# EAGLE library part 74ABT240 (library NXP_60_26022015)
Octal BUFFER and LINE DRIVER, 3-state
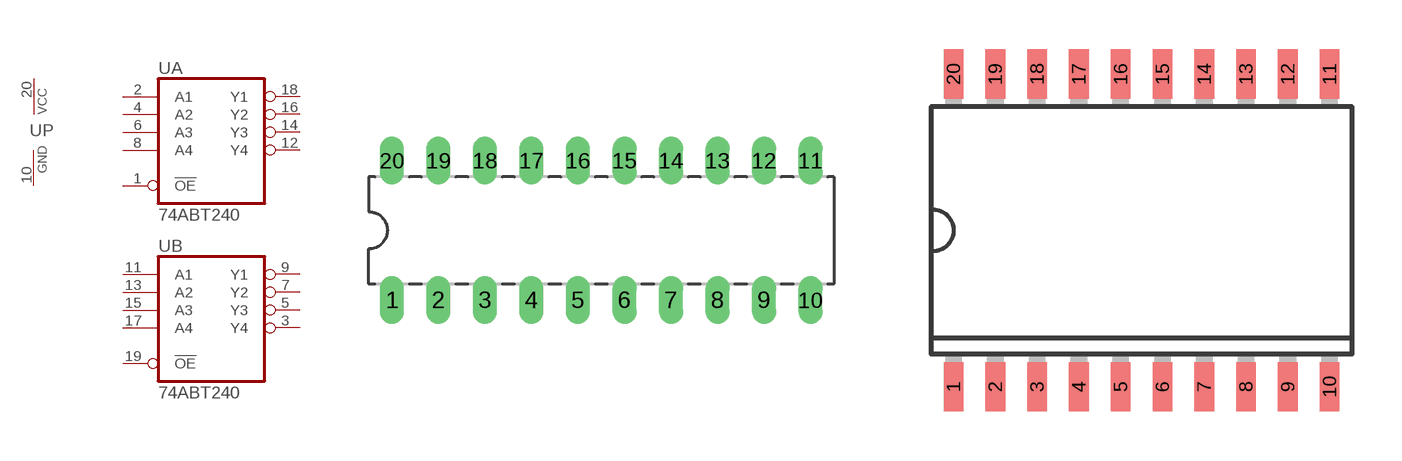
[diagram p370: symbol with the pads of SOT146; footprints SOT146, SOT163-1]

Designator prefix U; gates A=74240 B=74240 P=PWRN-3

## 74ABT240N  [SOT146]
1  A:!OE  in
2  A:A1  in
3  B:Y4  hiz
4  A:A2  in
5  B:Y3  hiz
6  A:A3  in
7  B:Y2  hiz
8  A:A4  in
9  B:Y1  hiz
10  P:GND  pwr
11  B:A1  in
12  A:Y4  hiz
13  B:A2  in
14  A:Y3  hiz
15  B:A3  in
16  A:Y2  hiz
17  B:A4  in
18  A:Y1  hiz
19  B:!OE  in
20  P:VCC  pwr

## 74ABT240D  [SOT163-1]
Pads as for SOT146

## 74ABT240DB  [SOT339]
Pads as for SOT146

## 74ABT240PW  [SOT360]
Pads as for SOT146

## Footprint SOT146 (pad centres in mm)
SOT146 DIP20: plastic dual in-line package; 20 leads (300 mil) JEDEC: MS-001 IEC: -- JEITA: SC-603
drill 0.813 long: 1 -11.43,-3.81; 2 -8.89,-3.81; 3 -6.35,-3.81; 4 -3.81,-3.81; 5 -1.27,-3.81; 6 1.27,-3.81; 7 3.81,-3.81; 8 6.35,-3.81; 9 8.89,-3.81; 10 11.43,-3.81; 11 11.43,3.81; 12 8.89,3.81; 13 6.35,3.81; 14 3.81,3.81; 15 1.27,3.81; 16 -1.27,3.81; 17 -3.81,3.81; 18 -6.35,3.81; 19 -8.89,3.81; 20 -11.43,3.81

## Footprint SOT163-1 (pad centres in mm)
SOT163-1 SO20: plastic small outline package; 20 leads; body width 7.5 mm JEDEC: MS-013 IEC: 075E04
smd 0.6 x 1.5: 1 -5.715,-4.75; 2 -4.445,-4.75; 3 -3.175,-4.75; 4 -1.905,-4.75; 5 -0.635,-4.75; 6 0.635,-4.75; 7 1.905,-4.75; 8 3.175,-4.75; 9 4.445,-4.75; 10 5.715,-4.75; 11 5.715,4.75; 12 4.445,4.75; 13 3.175,4.75; 14 1.905,4.75; 15 0.635,4.75; 16 -0.635,4.75; 17 -1.905,4.75; 18 -3.175,4.75; 19 -4.445,4.75; 20 -5.715,4.75

## Footprint SOT339 (pad centres in mm)
SOT339 SSOP20: plastic shrink small outline package; 20 leads; body width 5.3 mm JEDEC: MO-150 IEC: --
smd 0.4 x 1.1: 1 -2.925,-3.5; 2 -2.275,-3.5; 3 -1.625,-3.5; 4 -0.975,-3.5; 5 -0.325,-3.5; 6 0.325,-3.5; 7 0.975,-3.5; 8 1.625,-3.5; 9 2.275,-3.5; 10 2.925,-3.5; 11 2.925,3.5; 12 2.275,3.5; 13 1.625,3.5; 14 0.975,3.5; 15 0.325,3.5; 16 -0.325,3.5; 17 -0.975,3.5; 18 -1.625,3.5; 19 -2.275,3.5; 20 -2.925,3.5

## Footprint SOT360 (pad centres in mm)
SOT360 TSSOP20: plastic thin shrink small outline package; 20 leads; body width 4.4 mm JEDEC: MO-153 IEC:
smd 0.6 x 1.35: 1 -3.025,-2.925; 10 3.025,-2.925; 11 3.025,2.925; 20 -3.025,2.925
smd 0.4 x 1.35: 2 -2.275,-2.925; 3 -1.625,-2.925; 4 -0.975,-2.925; 5 -0.325,-2.925; 6 0.325,-2.925; 7 0.975,-2.925; 8 1.625,-2.925; 9 2.275,-2.925; 12 2.275,2.925; 13 1.625,2.925; 14 0.975,2.925; 15 0.325,2.925; 16 -0.325,2.925; 17 -0.975,2.925; 18 -1.625,2.925; 19 -2.275,2.925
